DATA_BLOCK DB98
TITLE =

AUTHOR:INA
FAMILY:StateMac
NAME:nb
VERSION:00.00


    FB98


BEGIN
       Write:=FALSE
       NodeID:=B#16#00
       Done:=FALSE
       Err:=FALSE
       ErrNo:=L#0
       xEdgeMerker:=FALSE
       xEdgeFlag:=FALSE
       xStep:=0
       xShutdown:=W#16#0006
       xEnableOperation:=W#16#000F

END_DATA_BLOCK
